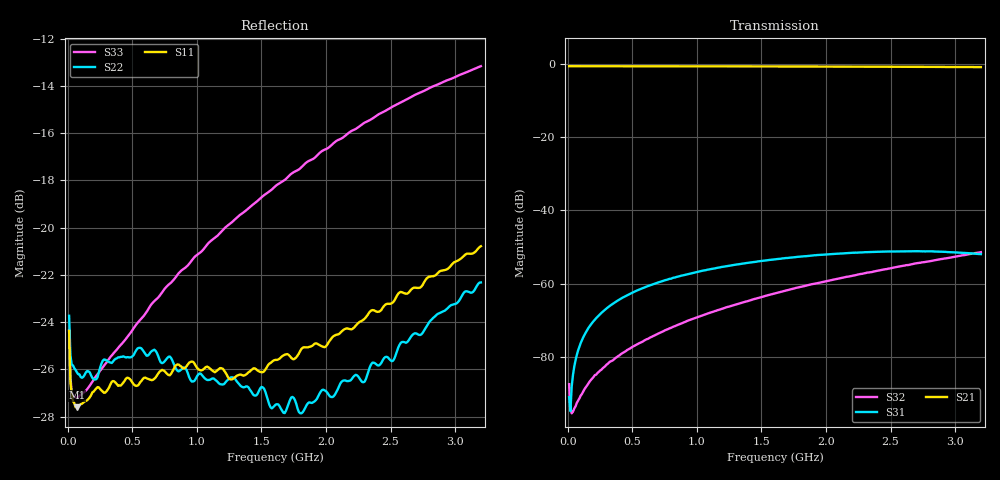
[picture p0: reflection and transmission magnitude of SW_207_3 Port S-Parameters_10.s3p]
! Created _Nov-02-2022_09-58-32
! Type : General
! Retest Level : 0
! Program : FASTESt Rev. 859
! DUT_TempC = 25.0
! Set_V1_Supply_V = 3.0
! V1_Supply_V = 3.002
! V1_Supply_I = -4e-06
! Set_V2_Supply_V = 0.0
! V2_Supply_V = -0.001
! V2_Supply_I = -5e-06
! RunID = 10
! SN = 5
! Comment = SW-207_SB5_RFc-RF1_room
! Input_Power = 5.0
! Measurement_Comment = None
! Freq	S11db	S11deg	S12db	S12deg	S13db	S13deg	S21db	S21deg	S22db	S22deg	S23db	S23deg	S31db	S31deg	S32db	S32deg	S33db	S33deg
# Hz S dB R 50
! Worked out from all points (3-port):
!   320 points, 10 MHz to 3.2 GHz, reference 50 ohm
!   strongest paths, dB at 10 MHz, 810 MHz, 1.61 GHz, 2.41 GHz, 3.2 GHz:
!     S21: -0.6, -0.6, -0.7, -0.7, -0.8
!     S31: -91.0, -58.5, -53.3, -51.3, -51.9
!     S32: -87.5, -71.9, -62.6, -56.4, -51.4
!   lowest |S11| = -27.6 dB at 70 MHz (marker M1), VSWR 1.09, Z = 54.2 - j0.979 ohm
!   |S11| at or under -10 dB: start of sweep to end of sweep
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1e7  -24.37 -43.0  -0.59 1.3  -90.73 -122.9
     -0.59 1.3  -23.73 -39.4  -87.16 -112.0
     -91.02 -125.1  -87.48 -111.5  -24.35 -37.8
7e7  -27.60 -12.5  -0.60 -6.0  -79.49 79.8
     -0.60 -6.0  -26.12 -11.2  -92.84 -95.6
     -79.45 80.0  -92.56 -94.8  -27.19 -6.4
3.1e8  -26.85 -16.8  -0.62 -27.4  -66.50 63.1
       -0.61 -27.5  -25.66 -17.2  -82.04 -139.0
       -66.50 62.9  -81.89 -138.5  -25.63 1.2
8.8e8  -25.89 -69.7  -0.63 -77.2  -57.85 18.4
       -0.63 -77.3  -26.01 -66.3  -70.94 150.3
       -57.81 18.1  -70.88 150.8  -21.81 -21.3
1.23e9  -26.21 -112.0  -0.65 -107.8  -55.28 -9.2
        -0.65 -107.8  -26.49 -107.7  -66.51 114.8
        -55.26 -9.3  -66.44 114.9  -19.95 -45.2
1.61e9  -25.60 -161.2  -0.67 -140.9  -53.39 -39.1
        -0.67 -140.9  -27.49 -158.3  -62.67 81.0
        -53.34 -39.2  -62.62 81.2  -18.24 -74.6
1.97e9  -25.03 150.6  -0.70 -172.2  -52.15 -67.4
        -0.70 -172.3  -26.87 150.3  -59.62 50.7
        -52.12 -67.6  -59.58 50.7  -16.76 -103.8
2.32e9  -23.72 108.9  -0.74 157.3  -51.42 -95.0
        -0.73 157.2  -26.24 100.4  -57.07 23.0
        -51.40 -95.2  -56.98 22.9  -15.50 -132.7
2.78e9  -22.15 56.6  -0.79 117.2  -51.22 -130.9
        -0.79 117.1  -24.18 46.3  -54.08 -11.6
        -51.18 -131.0  -54.00 -12.0  -14.15 -171.4
3.2e9  -20.79 10.2  -0.85 80.5  -51.97 -161.4
       -0.84 80.4  -22.32 3.3  -51.43 -41.6
       -51.95 -161.7  -51.42 -41.7  -13.17 152.2
